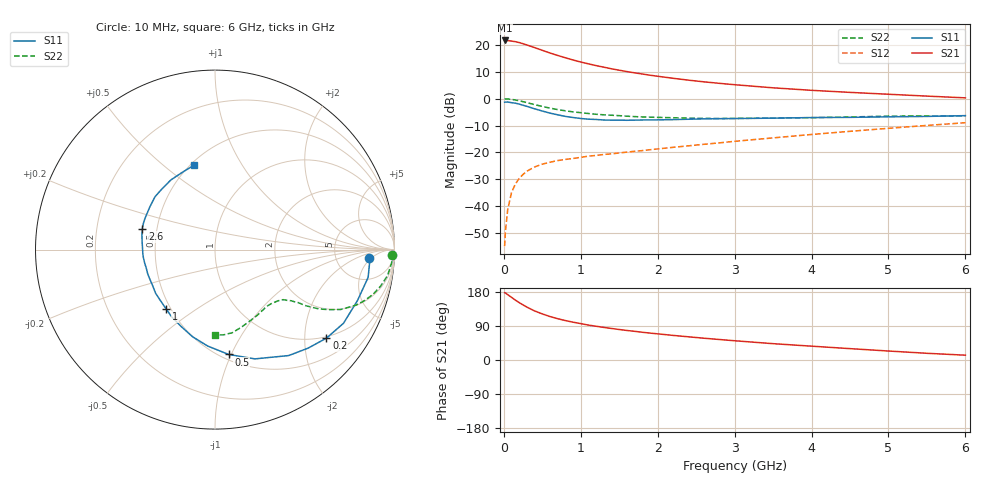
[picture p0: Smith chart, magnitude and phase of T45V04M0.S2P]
! Infineon Technologies  Discrete & RF Semiconductors
! BFR182T
! Si NPN RF Bipolar Junction Transistor in SC75
! VCE = 5 V  IC = 4 mA
! Common Emitter S-Parameters:  October  1999
# GHz  S  MA  R  50
!  f  S11  S21  S12  S22
! GHz  MAG  ANG  MAG  ANG  MAG  ANG  MAG  ANG
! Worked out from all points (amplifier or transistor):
!   36 points, 10 MHz to 6 GHz, reference 50 ohm
!   highest |S21| = 21.7 dB at 10 MHz (marker M1)
!   |S21| within 3 dB of that: start of sweep to 433.7 MHz
!   unconditionally stable (mu >= 1): 1.578 GHz to 4.126 GHz
!   at 250 MHz: K = 0.24, MSG = 24.3 dB, |S12| = -28.2 dB
!   at 1.4 GHz: K = 0.95, MSG = 15.8 dB, |S12| = -20.5 dB
!   at 6 GHz: K = 0.84, MSG = 4.6 dB, |S12| = -8.9 dB
!   S11 on the Smith chart (normalised r, x): 10 MHz: 12, -4; 200 MHz: 0.96, -2.55; 500 MHz: 0.55, -0.98; 1 GHz: 0.47, -0.38; 2.6 GHz: 0.41, +0.12; 6 GHz: 0.52, +0.64
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0.01  0.8605 -3.2  12.12 177.6  0.0018 87.0  0.9845 -1.6
0.02  0.8657 -2.7  12.02 177.2  0.0033 88.9  0.993 -1.7
0.05  0.8671 -10.3  12.09 172.4  0.0086 88.9  0.9866 -4.4
0.1  0.8429 -19.7  11.8 165.4  0.018 81.8  0.972 -8.6
0.15  0.8253 -29.8  11.51 158.0  0.0258 74.5  0.9442 -12.5
0.2  0.793 -38.5  11.07 151.4  0.0329 72.4  0.9144 -15.9
0.25  0.755 -46.7  10.53 145.3  0.039 66.6  0.8793 -18.9
0.3  0.719 -55.2  9.989 139.6  0.0448 64.0  0.8446 -21.5
0.4  0.6483 -69.9  8.929 129.5  0.0536 58.0  0.7755 -25.5
0.5  0.589 -82.6  7.942 121.6  0.0605 54.8  0.717 -27.8
0.6  0.539 -94.3  7.083 114.7  0.0657 52.3  0.6676 -29.7
0.7  0.5011 -104.5  6.378 109.0  0.0706 51.3  0.6271 -30.8
0.8  0.4682 -113.7  5.776 104.0  0.0741 50.3  0.5949 -31.7
1  0.4284 -129.4  4.811 96.0  0.0811 50.0  0.5493 -32.5
1.1  0.4155 -137.5  4.45 92.1  0.0852 50.4  0.5294 -33.3
1.6  0.3966 -165.1  3.194 77.9  0.1014 52.8  0.4724 -36.2
2.2  0.4081 174.2  2.397 64.9  0.1244 56.5  0.4421 -41.7
2.6  0.4212 164.0  2.06 57.5  0.1416 58.4  0.43 -46.2
3.5  0.4342 146.6  1.593 43.1  0.1865 60.1  0.4354 -57.5
4.5  0.4492 131.1  1.31 30.0  0.247 58.7  0.457 -71.4
5.5  0.4677 112.8  1.117 17.7  0.3181 54.9  0.4773 -84.2
6  0.4839 104.1  1.036 12.7  0.357 51.8  0.4761 -89.7
